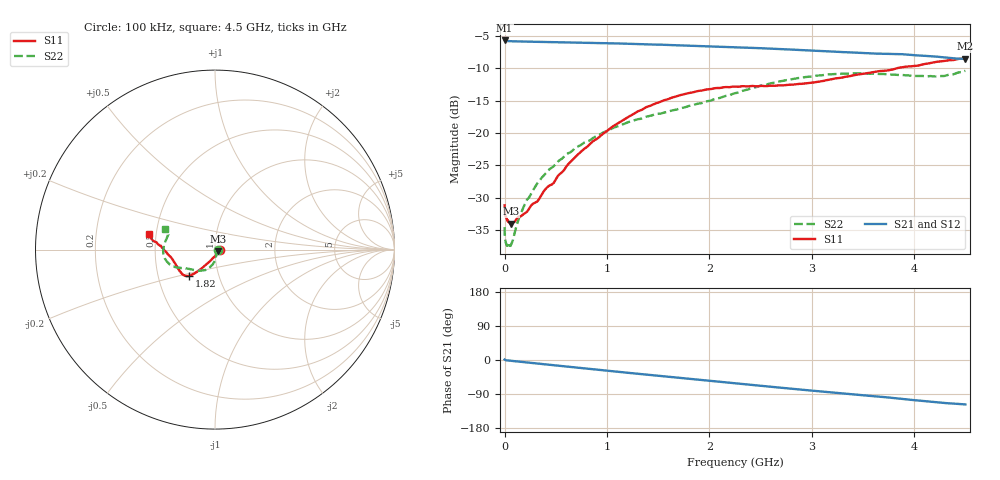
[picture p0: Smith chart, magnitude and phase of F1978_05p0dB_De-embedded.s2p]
! Integrated Device Technology
! Corporate Headquarters
! 6024 Silver Creek Valley Road
! San Jose, CA 95138  USA
! Phone:  1-408-284-8200
! Toll Free:  1-800-223-1366
! Webpage:  http://www.idt.com/
! Timing and RF Division
! 515 Groton Road, Suite 102
! Westford, MA 01886-6024
! Device:  F1978
! Description: 6-bit, 75 ohm, 0.5 dB Digital Step Attenuator
! Frequency:  5.0 MHz -  3.00 GHz
! Package:  4x4 mm QFN Plastic Package: 20 pin
! Ports:  2 RF, 11 DC
!  Pin  1  = D5 (16 dB)
!  Pin  2  = RF1  =  Port 1
!  Pin  3  = Serial Data In (DATA)
!  Pin  4  = Serial Clock (CLK)
!  Pin  5  = Serial Latch Enable (LE)
!  Pin  6  = VDD
!  Pin  7  = NC
!  Pin  8  = NC
!  Pin  9  = NC
!  Pin 10  = GND
!  Pin 11  = GND
!  Pin 12  = NC
!  Pin 13  = VMODE
!  Pin 14  = RF2  =  Port 2
!  Pin 15  = D4 (8 dB)
!  Pin 16  = D3 (4 dB)
!  Pin 17  = D2 (2 dB)
!  Pin 18  = NC
!  Pin 19  = D1 (1 dB)
!  Pin 20  = D0 (0.5 dB)
! State:  10
! Atten State:  5.0 dB
! Voltage:  +3.30 Volts
! Current:  0.594 mA
! Data:  The device was measured on a F1975 evaluation board which has
!  individual transmission lines to the RF pins.  Data was collected
!  using a calibrated network analyzer.  The evaluation board was
!  de-embedded using Automatic Fixture Removal (AFR).
!  The reference plane is the edge of the package pin.
! Misc:
!  Action Tracker AT0416
! Date Measured:  2018-02-08
! Date:  2018-03-26  MJV
! Note:
!  Integrated Device Technology supplies this data as a sample of measured
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# GHz S dB R 75
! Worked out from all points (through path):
!   291 points, 100 kHz to 4.5 GHz, reference 75 ohm
!   highest |S21| = -5.70 dB at 100 kHz (marker M1); lowest = -8.5 dB at 4.5 GHz (marker M2)
!   group delay of S21, straight-line fit = 73.4 ps
!   lowest |S11| = -34.0 dB at 60 MHz (marker M3), VSWR 1.04, Z = 77.8 - j1.3 ohm
!   |S11| at or under -10 dB: start of sweep to 3.831 GHz
!   |S22| runs from -37.5 to -10.4 dB; largest |S21 - S12| = 0.00018
!   S11 on the Smith chart (normalised r, x): 100 kHz: 1.06, +0.00; 1.82 GHz: 0.72, -0.22; 4.5 GHz: 0.46, +0.09
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0.0001  -31.19 0.1  -5.70 1.2  -5.70 1.2  -34.54 0.3
0.0009  -32.00 -3.1  -5.73 1.0  -5.73 1.0  -35.61 -2.9
0.003  -32.40 -3.2  -5.75 0.7  -5.75 0.7  -36.23 -4.4
0.013  -32.99 -9.1  -5.78 -0.6  -5.78 -0.6  -37.03 -14.5
0.06  -33.99 -24.8  -5.82 -2.0  -5.82 -2.0  -37.36 -42.5
0.08  -33.90 -32.6  -5.83 -2.6  -5.83 -2.6  -36.62 -54.5
0.12  -33.20 -42.6  -5.85 -3.7  -5.85 -3.7  -34.12 -65.9
0.18  -32.60 -53.5  -5.87 -5.5  -5.87 -5.5  -31.63 -72.7
0.32  -30.57 -78.1  -5.91 -9.4  -5.91 -9.4  -27.76 -82.4
0.4  -28.64 -88.8  -5.93 -11.6  -5.93 -11.6  -26.25 -85.1
0.48  -27.71 -97.0  -5.96 -13.8  -5.96 -13.8  -25.13 -88.7
0.52  -26.64 -101.2  -5.97 -14.9  -5.97 -14.9  -24.42 -90.4
0.76  -22.69 -114.3  -6.04 -21.5  -6.04 -21.5  -21.69 -98.6
1.08  -18.75 -123.5  -6.15 -30.4  -6.15 -30.4  -19.10 -108.8
1.52  -15.19 -130.6  -6.35 -42.2  -6.35 -42.2  -17.00 -124.1
1.82  -13.77 -134.4  -6.52 -50.1  -6.52 -50.1  -15.76 -135.6
2.26  -12.83 -143.5  -6.75 -61.7  -6.74 -61.7  -13.81 -149.4
2.68  -12.63 -157.4  -7.02 -72.7  -7.02 -72.7  -12.04 -157.8
3.02  -12.19 -168.7  -7.28 -81.3  -7.27 -81.3  -11.21 -165.8
3.76  -10.28 175.8  -7.78 -99.2  -7.78 -99.2  -10.96 173.8
4.22  -9.00 171.1  -8.20 -111.5  -8.20 -111.5  -11.27 162.2
4.5  -8.51 166.8  -8.54 -117.2  -8.53 -117.2  -10.38 158.0
